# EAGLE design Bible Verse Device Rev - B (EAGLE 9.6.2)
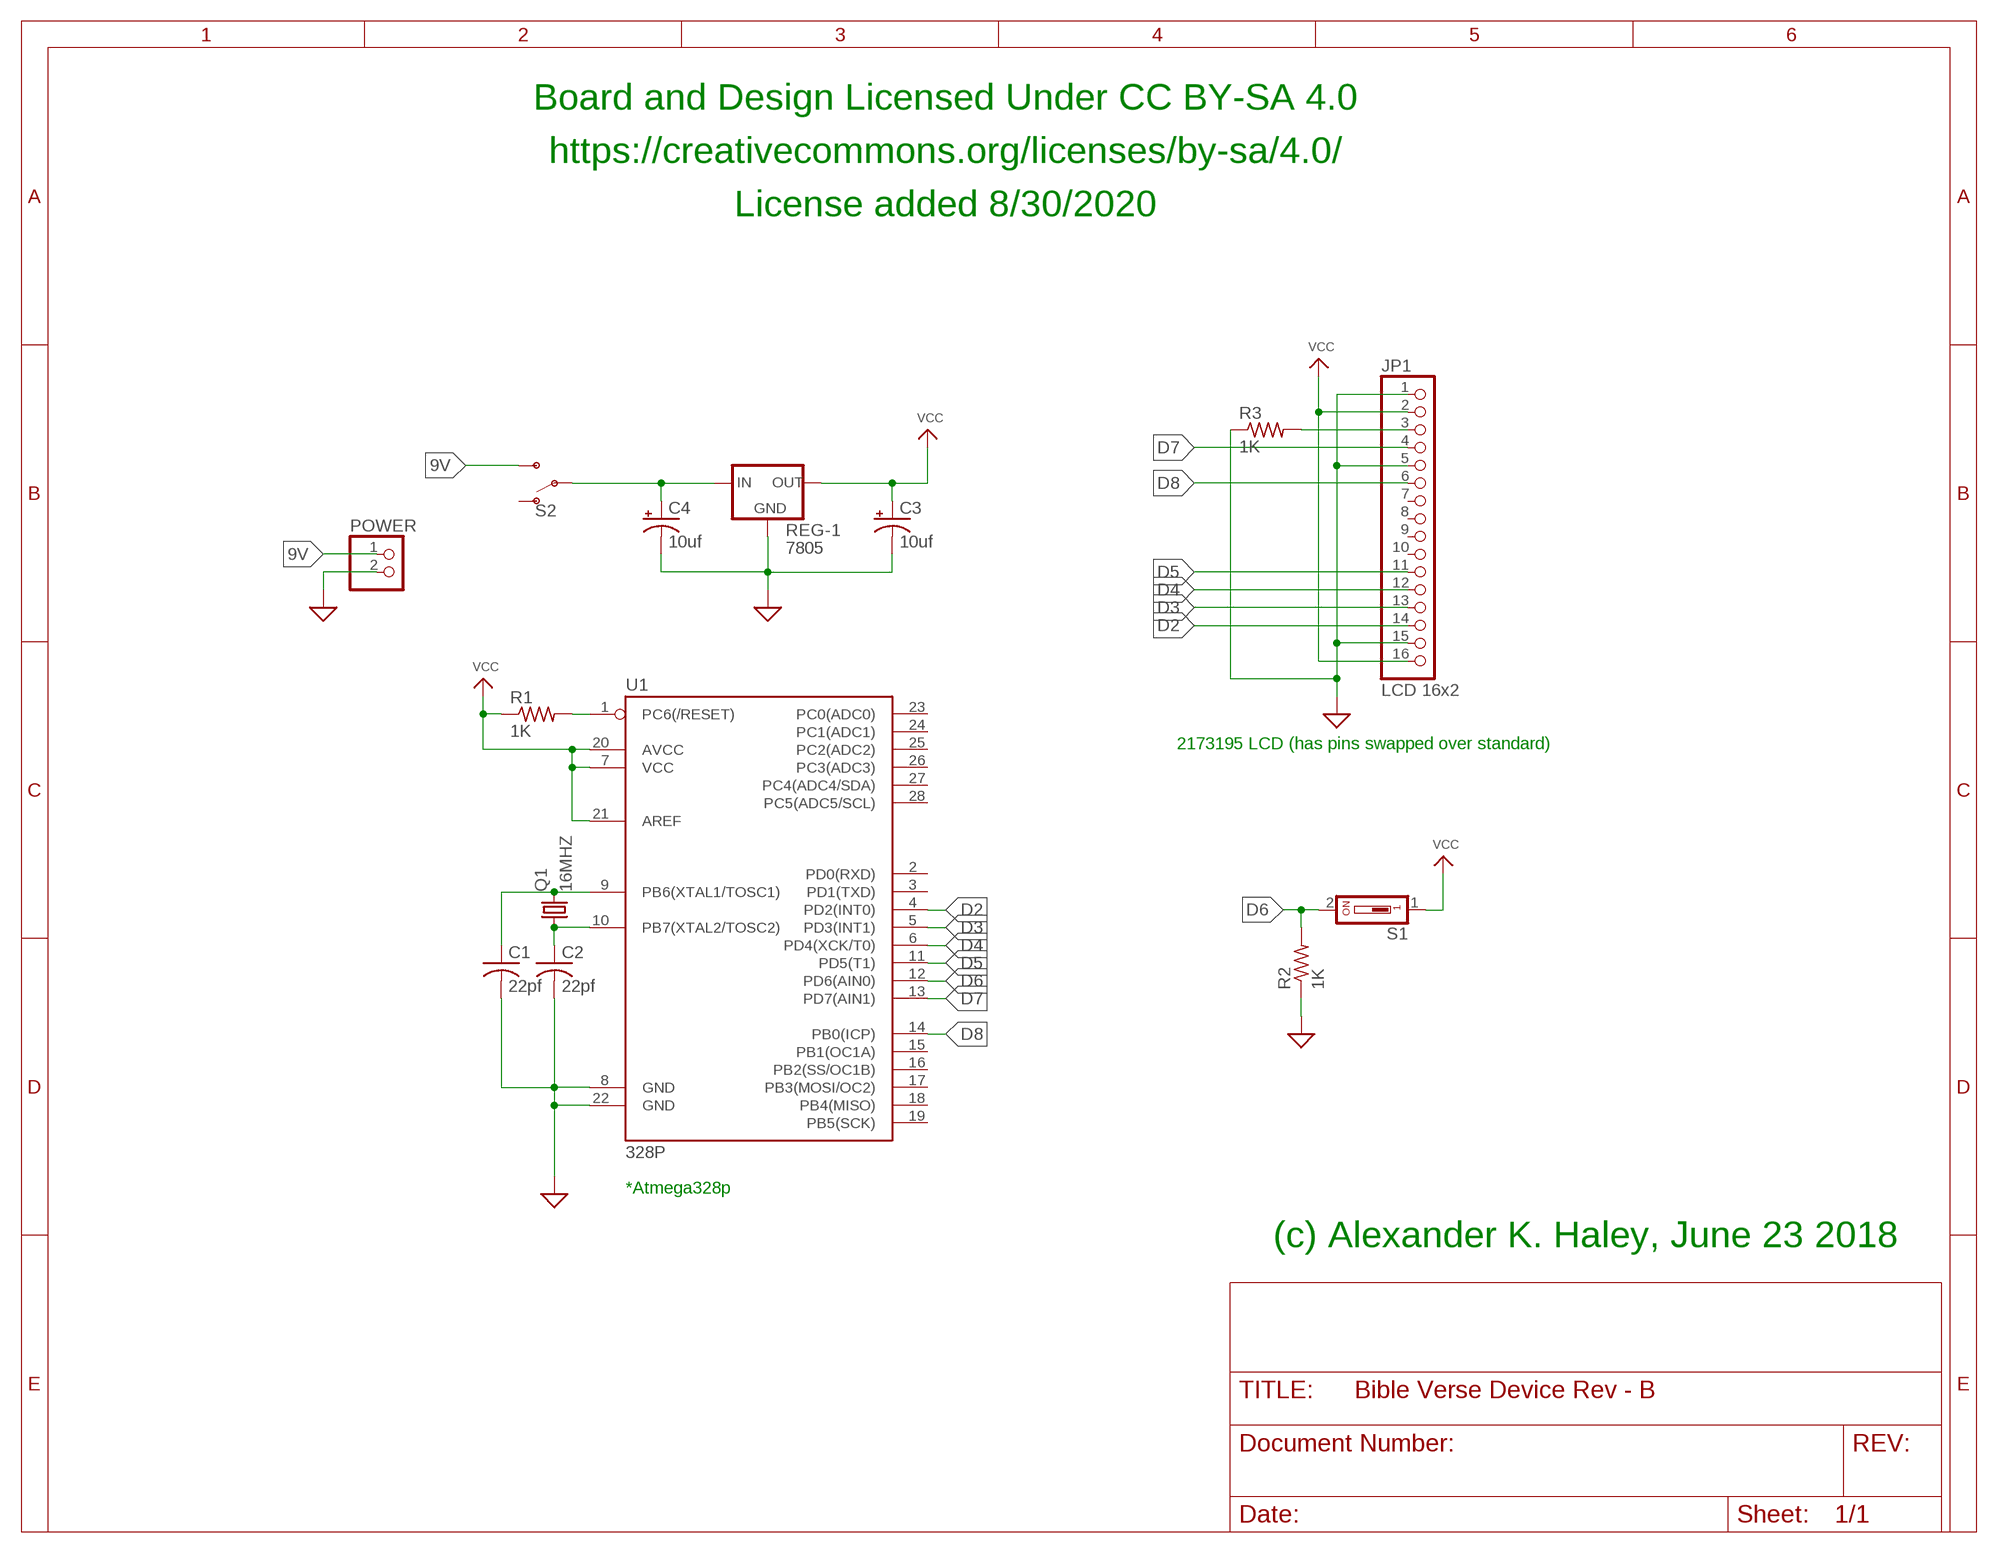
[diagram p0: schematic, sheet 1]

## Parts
C1  22pf  C-US025-025X050  [C025-025X050]
C2  22pf  C-US025-025X050  [C025-025X050]
C3  10uf  CPOL-USE2.5-6  [E2,5-6]
C4  10uf  CPOL-USE2.5-6  [E2,5-6]
JP1  LCD 16x2  PINHD-1X16  [1X16]
POWER  PINHD-1X2  [1X02]
Q1  16MHZ  CRYSTALHC49S  [HC49/S]
R1  1K  R-US_0207/10  [0207/10]
R2  1K  R-US_0207/10  [0207/10]
R3  1K  R-US_0207/10  [0207/10]
REG-1  7805  V_REG_78XX-TO-220  [TO-220-ALT]
S1  SD4-01  [SD4-01]
S2  SWITCH-SPDT-PTH-11.6X4.0MM-LOCK  [SWITCH_SPDT_PTH_11.6X4.0MM_LOCK]
U1  328P  ATMEGA328P_PDIP  [DIP28]

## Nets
9V: POWER.1 S2.3(S)
D2: JP1.14 U1.4(PD2(INT0))
D3: JP1.13 U1.5(PD3(INT1))
D4: JP1.12 U1.6(PD4(XCK/T0))
D5: JP1.11 U1.11(PD5(T1))
D6: R2.2 S1.2 U1.12(PD6(AIN0))
D7: JP1.4 U1.13(PD7(AIN1))
D8: JP1.6 U1.14(PB0(ICP))
GND: C1.2 C2.2 C3.- C4.- JP1.1 JP1.5 JP1.15 POWER.2 R2.1 R3.1 REG-1.GND U1.8(GND) U1.22(GND) ; supply symbol labelled SUP
N$1: C1.1 Q1.2 U1.9(PB6(XTAL1/TOSC1))
N$2: C2.1 Q1.1 U1.10(PB7(XTAL2/TOSC2))
N$3: R1.2 U1.1(PC6(/RESET))
N$4: C4.+ REG-1.IN S2.2(P)
N$8: JP1.3 R3.2
VCC: C3.+ JP1.2 JP1.16 R1.1 REG-1.OUT S1.1 U1.7(VCC) U1.20(AVCC) U1.21(AREF)
Unconnected: JP1.7 JP1.8 JP1.9 JP1.10 S2.1(O) U1.2(PD0(RXD)) U1.3(PD1(TXD)) U1.15(PB1(OC1A)) U1.16(PB2(SS/OC1B)) U1.17(PB3(MOSI/OC2)) U1.18(PB4(MISO)) U1.19(PB5(SCK)) U1.23(PC0(ADC0)) U1.24(PC1(ADC1)) U1.25(PC2(ADC2)) U1.26(PC3(ADC3)) U1.27(PC4(ADC4/SDA)) U1.28(PC5(ADC5/SCL))

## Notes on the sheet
- Board and Design Licensed Under CC BY-SA 4.0
- https://creativecommons.org/licenses/by-sa/4.0/
- License added 8/30/2020
- 2173195 LCD (has pins swapped over standard)
- *Atmega328p
- (c) Alexander K. Haley, June 23 2018

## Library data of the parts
C1 C2 = resistor:C-US: CAPACITOR, American symbol
C3 C4 = rcl:CPOL-US: POLARIZED CAPACITOR, American symbol; SPICEPREFIX: C
JP1 = pinhead:PINHD-1X16: PIN HEADER
POWER = pinhead:PINHD-1X2: PIN HEADER
Q1 = crystal:CRYSTAL: CRYSTAL; OC_FARNELL: 1667008; OC_NEWARK: unknown
R1 R2 = rcl:R-US_: RESISTOR, American symbol; SPICEPREFIX: R
R3 = resistor:R-US_: RESISTOR, American symbol
REG-1 = SparkFun-IC-Power:V_REG_78XX: Voltage Regulator Standard 78xx regulator. IGO (Input Ground Output). Spark Fun Electronics SKU : COM-00107; PROD_ID: VREG-08450; SF_ID: COM-00107
S1 = switch-dil:SD4-01: DIL/CODE SWITCH; OC_FARNELL: unknown; OC_NEWARK: unknown
S2 = SparkFun-Switches:SWITCH-SPDT: Single Pole, Double Throw (SPDT) Switch Single-pole, double-throw (SPDT) switch. Variant Overview SMD-AYZ0202 Surface Mount DPDT Switch (COM-00597) Used on e.g. LilyPad Arduino USB - ATmega32U4 Board PTH-11.6X4.0MM SPDT Mini Power Switch (COM-00102) Used on e.g. SparkFun Simon Says - Through-Hole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; PROD_ID: SWCH-08261; SF_SKU: COM-00102
U1 = SparkFun-IC-Microcontroller:ATMEGA328P_PDIP: Atmel 328P Through hole ATMEGA328P uC used in the Arduino 32kb flash, 1k EEPROM, 2k SRAM Datasheet SparkFun Products Storefront component: AVR 28 Pin 20MHz 32K 6A/D - ATMega328P (COM-09061) SparkFun Simon Says - Through-Hole Soldering Kit (KIT-10547) SparkFun Learn to Solder - Simon Says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; PROD_ID: IC-09136

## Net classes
0 default: width 0.254 mm, clearance 0.254 mm

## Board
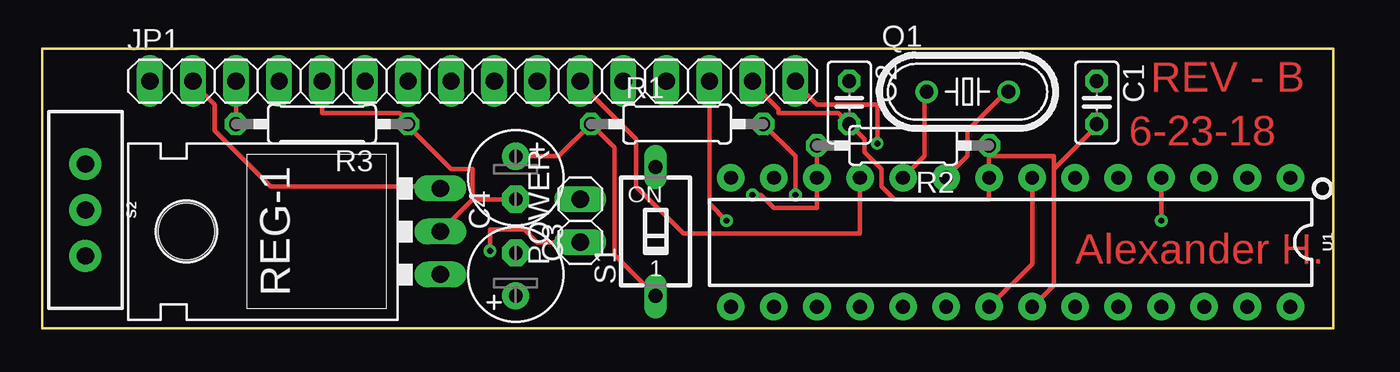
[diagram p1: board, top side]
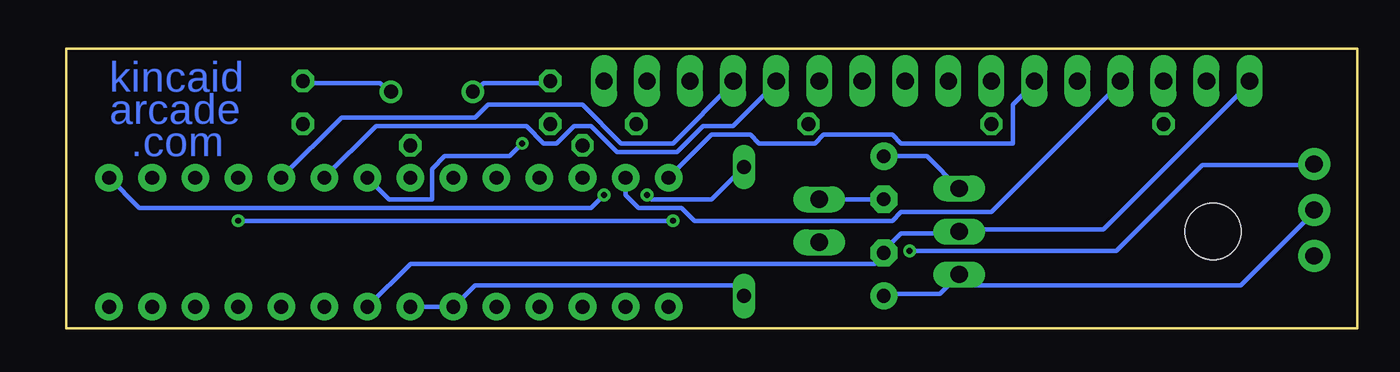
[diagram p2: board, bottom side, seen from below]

Size 76.2 x 16.51 mm. Coordinates in mm from the lower left corner, seen from the top.
Outline: 0,16.51 76.2,16.51 76.2,0 0,0 0,16.51
Copper layers (1*16): Top 0.035mm / dielectric 1.5mm / Bottom 0.035mm
Design rules "default": minimum track width 6mil, minimum drill 0.35mm, track to track 6mil, track to pad 6mil, pad to pad 6mil, via to via 6mil, smd to smd 6mil, copper to edge 40mil, drill to drill 6mil, minimum pad ring 10mil, minimum via ring 8mil, stop-mask expansion 4mil, vias tented up to drill 0mil, thermal gap 10mil

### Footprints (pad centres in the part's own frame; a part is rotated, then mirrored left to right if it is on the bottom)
C025-025X050 = drill 0.813 octagon: 1 -1.27,0; 2 1.27,0
E2,5-6 = drill 0.813 pad 1.6: + -1.27,0 | drill 0.813 pad 1.6 octagon: - 1.27,0
1X16 = drill 1.016 long: 1 -19.05,0; 2 -16.51,0; 3 -13.97,0; 4 -11.43,0; 5 -8.89,0; 6 -6.35,0; 7 -3.81,0; 8 -1.27,0; 9 1.27,0; 10 3.81,0; 11 6.35,0; 12 8.89,0; 13 11.43,0; 14 13.97,0; 15 16.51,0; 16 19.05,0
1X02 = drill 1.016 long: 1 -1.27,0; 2 1.27,0
HC49/S = drill 0.813: 1 -2.413,0; 2 2.413,0
0207/10 = drill 0.813 octagon: 1 -5.08,0; 2 5.08,0
TO-220-ALT = drill 1.016 long: GND 0,-3.81; IN -2.54,-3.81; OUT 2.54,-3.81 | hole 3.302: 0,11.176
SD4-01 = drill 0.813 long: 1 0,-3.81; 2 0,3.81
SWITCH_SPDT_PTH_11.6X4.0MM_LOCK = drill 1.016 pad 1.88: 1 0,2.718; 2 0,0; 3 0,-2.718
DIP28 = drill 0.813 pad 1.626: 1 -16.51,-3.81; 2 -13.97,-3.81; 3 -11.43,-3.81; 4 -8.89,-3.81; 5 -6.35,-3.81; 6 -3.81,-3.81; 7 -1.27,-3.81; 8 1.27,-3.81; 9 3.81,-3.81; 10 6.35,-3.81; 11 8.89,-3.81; 12 11.43,-3.81; 13 13.97,-3.81; 14 16.51,-3.81; 15 16.51,3.81; 16 13.97,3.81; 17 11.43,3.81; 18 8.89,3.81; 19 6.35,3.81; 20 3.81,3.81; 21 1.27,3.81; 22 -1.27,3.81; 23 -3.81,3.81; 24 -6.35,3.81; 25 -8.89,3.81; 26 -11.43,3.81; 27 -13.97,3.81; 28 -16.51,3.81

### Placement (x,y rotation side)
C1  62.23,13.34 270 top
C2  47.62,13.34 270 top
C3  27.94,8.89 270 top
C4  27.94,3.18 90 top
JP1  25.4,14.61 0 top
POWER  31.75,6.35 90 top
Q1  54.61,13.97 0 top
R1  37.47,12.07 0 top
R2  50.8,10.8 180 top
R3  16.51,12.07 180 top
REG-1  19.69,5.72 90 top
S1  36.19,5.72 0 top
S2  2.54,6.99 180 top
U1  57.15,5.08 180 top

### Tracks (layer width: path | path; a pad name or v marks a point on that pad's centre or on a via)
9V  (via drill 0.35)
  Top 0.254: POWER.1 29.21,5.08 28.45,5.84 26.42,5.84 v26.42,4.57
  Bottom 0.254: v26.42,4.57 14.22,4.57 9.14,9.65 2.54,9.65 S2.3
D2  (via drill 0.35)
  Top 0.254: JP1.14 39.37,7.37 v40.39,6.35 | U1.4 v66.04,6.35
  Bottom 0.254: v66.04,6.35 v40.39,6.35
D3
  Bottom 0.254: U1.5 59.94,12.45 52.07,12.45 51.31,13.21 45.72,13.21 43.43,10.92 40.39,10.92 36.83,14.48 JP1.13
D4
  Bottom 0.254: U1.6 57.91,11.94 49.02,11.94 48.01,10.92 47.24,10.92 46.23,11.94 45.21,11.94 43.69,10.41 40.13,10.41 38.61,11.94 36.83,11.94 34.29,14.48 JP1.12
D5
  Top 0.254: U1.11 48.26,5.59 37.85,5.59 35.05,8.38 35.05,11.18 31.75,14.48 JP1.11
D6  (via drill 0.35)
  Top 0.254: v41.91,7.87 42.42,7.87 43.18,7.11 45.72,7.11 U1.12 R2.2
  Bottom 0.254: S1.2 38.1,7.62 41.66,7.62 v41.91,7.87
D7
  Bottom 0.254: U1.13 43.18,7.87 42.42,7.11 39.88,7.11 39.12,6.35 27.43,6.35 26.92,6.86 21.59,6.86 13.97,14.48 JP1.4
D8
  Bottom 0.254: U1.14 38.1,11.43 35.81,11.43 35.31,10.92 32,10.92 31.5,11.43 27.43,11.43 26.92,10.92 20.32,10.92 20.32,13.21 19.05,14.48 JP1.6
GND
  Top 0.254: JP1.15 41.91,14.48 43.43,12.95 43.43,12.7 46.99,12.7 C2.2 48.51,11.18 48.51,10.41 49.53,9.4 49.53,8.38 50.29,7.62 55.88,7.62 U1.8 55.88,10.16 | 55.88,10.16 R2.1 55.88,10.67 | 59.69,9.4 62.23,11.94 C1.2 | 59.69,9.4 59.69,2.54 U1.22 | 55.88,10.16 59.69,10.16 59.69,9.4 | JP1.5 16.51,12.7 21.08,12.7 21.59,12.19 R3.1 21.59,11.94 24.13,9.4 25.4,9.4 25.4,7.62 | 25.4,7.62 C3.- | REG-1.GND 25.4,7.62
  Bottom 0.254: C3.- POWER.2 | JP1.1 6.35,14.48 14.99,5.84 23.37,5.84 REG-1.GND 23.62,5.59 26.92,5.59 27.94,4.57 C4.- 27.94,4.32 28.45,3.81 55.88,3.81 U1.22
N$1
  Top 0.254: U1.9 54.61,10.16 54.61,11.68 56.9,13.97 Q1.2
  Bottom 0.254: Q1.2 57.15,13.97 57.66,14.48 62.23,14.48 C1.1
N$2
  Top 0.254: U1.10 52.07,10.16 52.07,13.97 Q1.1
  Bottom 0.254: Q1.1 52.07,13.97 51.56,14.48 47.75,14.48 C2.1
N$3  (via drill 0.35)
  Top 0.254: R1.2 44.45,10.16 v44.45,7.87
  Bottom 0.254: v44.45,7.87 45.21,7.11 71.88,7.11 U1.1
N$4
  Bottom 0.254: 24.13,2.54 24.64,2.03 27.94,2.03 C4.+ | 24.13,2.54 REG-1.IN 23.62,3.05 | 24.13,2.54 6.86,2.54 2.54,6.86 S2.2
N$8
  Top 0.254: JP1.3 R3.2
VCC  (via drill 0.35)
  Top 0.254: v49.28,10.92 49.28,13.21 45.72,13.21 44.45,14.48 JP1.16 | U1.21 58.42,3.81 U1.7 | C3.+ 30.48,10.16 R1.1 33.78,10.67 33.78,4.32 S1.1 | JP1.2 8.89,14.48 10.16,13.21 10.16,11.68 13.46,8.38 23.37,8.38 REG-1.OUT
  Bottom 0.254: U1.21 U1.20 52.07,2.54 36.83,2.54 S1.1 | v49.28,10.92 50.04,10.16 53.85,10.16 54.61,9.4 54.61,7.62 57.15,7.62 U1.7 | REG-1.OUT 25.4,10.16 C3.+

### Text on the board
Top: REV - B | 6-23-18 | Alexander H.
Bottom: kincaid | arcade | .com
